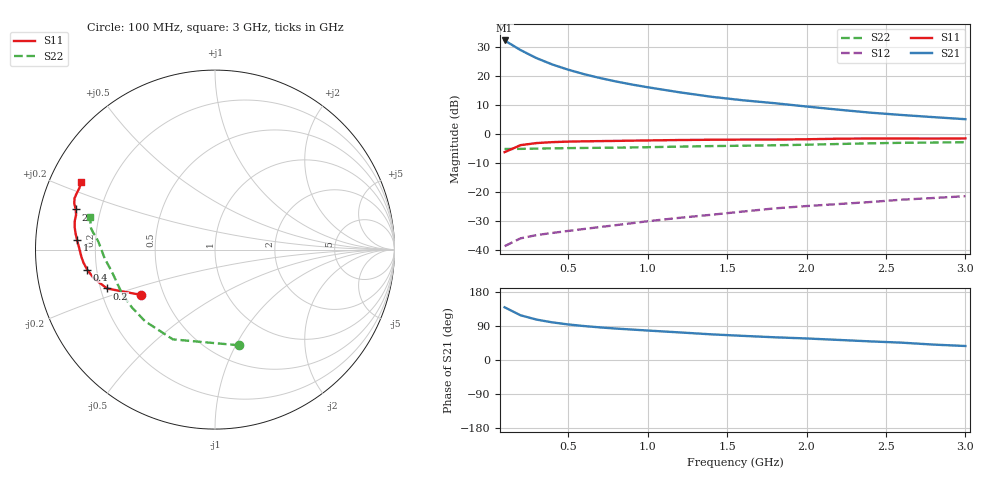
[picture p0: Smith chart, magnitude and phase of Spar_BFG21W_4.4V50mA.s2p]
! Filename: 4_450bfg21.001
! Title: BFG21W
! Bias: Vce=4.4V; Ic=50mA
! Company: NXP Semiconductors NL
! User: Quality&Reliability T&D
! Measure time: 10 Nov 1999 / 11:46:36
#  MHz  S  MA  R 50
! Freq  S11  S21  S12  S22  :
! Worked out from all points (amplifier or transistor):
!   20 points, 100 MHz to 3 GHz, reference 50 ohm
!   highest |S21| = 32.1 dB at 100 MHz (marker M1)
!   |S21| within 3 dB of that: start of sweep to 191 MHz
!   unconditionally stable (mu >= 1): 816.2 MHz to end of sweep
!   at 400 MHz: K = 0.74, MSG = 28.9 dB, |S12| = -34.0 dB
!   at 1.2 GHz: K = 1.08, MAG = 19.9 dB, |S12| = -28.8 dB
!   at 3 GHz: K = 1.05, MAG = 11.8 dB, |S12| = -21.4 dB
!   S11 on the Smith chart (normalised r, x): 100 MHz: 0.37, -0.24; 200 MHz: 0.23, -0.17; 400 MHz: 0.16, -0.08; 1 GHz: 0.13, +0.04; 2 GHz: 0.11, +0.14; 3 GHz: 0.10, +0.24
100  0.485 -148.7  40.21 139.1  0.01178 41.6  0.5497 -75.9
200  0.6396 -160.2  27.51 118.0  0.01605 38.5  0.5524 -115.1
300  0.6946 -166.8  20.04 106.7  0.01823 39.1  0.5579 -134.3
400  0.7209 -171.1  15.56 99.3  0.01988 41.8  0.5641 -145.2
500  0.7358 -174.2  12.65 93.8  0.02151 44.5  0.5691 -152.2
600  0.7448 -176.7  10.6 89.6  0.02325 47.7  0.5731 -157.0
700  0.7508 -178.8  9.108 86.0  0.0251 50.8  0.5763 -160.7
800  0.7568 179.3  7.951 83.0  0.02703 53.7  0.5797 -163.8
900  0.7642 177.5  7.045 80.4  0.02917 56.4  0.5845 -166.4
1000  0.7709 175.9  6.32 77.8  0.03157 58.4  0.5903 -168.7
1200  0.7835 173.1  5.179 72.8  0.03612 61.7  0.6038 -172.5
1400  0.7922 170.8  4.342 67.7  0.04076 64.0  0.6168 -175.5
1600  0.7974 168.4  3.776 63.7  0.04634 66.0  0.6257 -178.1
1800  0.7978 165.9  3.363 59.9  0.05251 67.4  0.6367 179.1
2000  0.8078 163.9  2.948 56.8  0.05753 68.8  0.6511 176.2
2200  0.8252 161.8  2.605 53.0  0.0623 69.5  0.6694 173.7
2400  0.8331 159.9  2.315 49.1  0.06748 69.4  0.6884 171.8
2600  0.8321 158.0  2.109 45.7  0.07408 68.9  0.7017 170.1
2800  0.8296 155.7  1.937 40.6  0.07917 67.7  0.7093 168.0
3000  0.8349 153.1  1.786 36.9  0.08506 67.1  0.719 165.3
